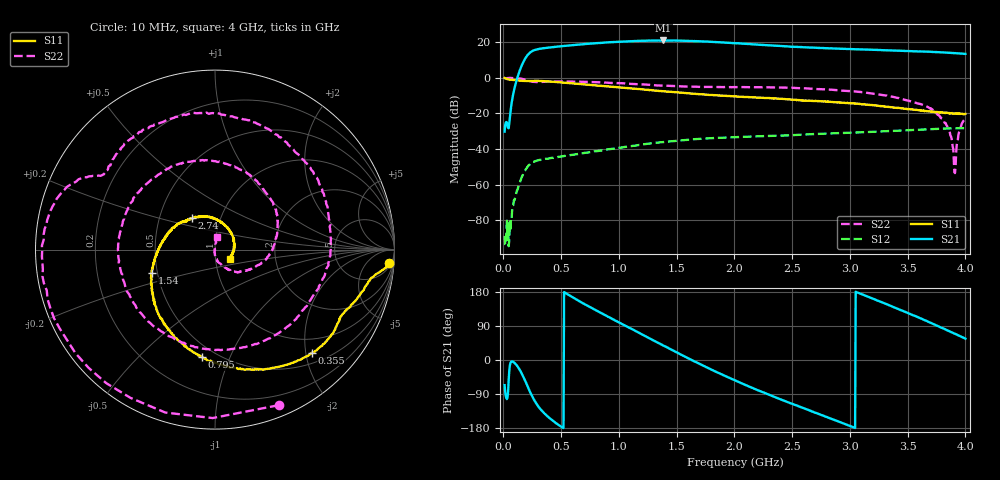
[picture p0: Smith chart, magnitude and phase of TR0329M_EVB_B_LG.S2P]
!Agilent Technologies,E5071C,MY46523237,B.13.01
!Date: Thu Jul 14 13:05:57 2022
!Data & Calibration Information:
!Freq	S11:SOLT2(ON)	S21:SOLT2(ON)	S12:SOLT2(ON)	S22:SOLT2(ON)
!PortZ  Port1:50+j0  Port2:50+j0
!Above PortZ is port z conversion or system Z0 setting when saving the data.
!When reading, reference impedance value at option line is always used.
# Hz S dB R 50
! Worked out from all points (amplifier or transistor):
!   799 points, 10 MHz to 4 GHz, reference 50 ohm
!   highest |S21| = 20.8 dB at 1.385 GHz (marker M1)
!   |S21| within 3 dB of that: 541.7 MHz to 2.374 GHz (1.832 GHz wide, 126 % of centre)
!   unconditionally stable (mu >= 1): start of sweep to end of sweep
!   at 675 MHz: K = 2.45, MAG = 23.8 dB, |S12| = -42.5 dB
!   at 2.005 GHz: K = 1.89, MAG = 20.9 dB, |S12| = -33.4 dB
!   at 4 GHz: K = 2.88, MAG = 13.3 dB, |S12| = -28.3 dB
!   S11 on the Smith chart (normalised r, x): 10 MHz: 9, -23; 355 MHz: 0.70, -2.13; 795 MHz: 0.42, -0.80; 1.54 GHz: 0.47, -0.14; 2.74 GHz: 0.73, +0.27; 4 GHz: 1.17, -0.12
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1e7  -0.25 -4.4  -30.33 -66.4  -88.77 103.1  -0.57 -67.8
1.25e8  -1.59 -20.0  0.84 -18.4  -62.16 -179.2  -0.45 171.6
1.95e8  -1.98 -26.9  11.34 -59.5  -51.30 142.2  -1.36 152.7
2.6e8  -1.90 -33.7  15.18 -102.3  -47.25 103.6  -2.44 146.8
3.55e8  -2.06 -46.6  16.48 -141.1  -45.68 72.9  -2.39 137.9
5.1e8  -2.78 -66.2  17.61 -178.0  -44.06 48.6  -2.22 117.2
6.75e8  -3.73 -84.5  18.60 152.0  -42.49 32.1  -2.42 92.6
7.95e8  -4.38 -96.8  19.20 132.1  -41.37 21.7  -2.61 73.6
1.09e9  -5.96 -124.4  20.31 84.7  -38.57 -4.9  -3.47 21.6
1.34e9  -7.46 -145.3  20.67 45.0  -36.43 -29.7  -4.45 -30.5
1.385e9  -7.70 -148.6  20.78 38.2  -36.19 -34.8  -4.51 -40.4
1.54e9  -8.50 -159.6  20.68 13.4  -35.21 -50.7  -4.94 -75.1
1.745e9  -9.53 -173.2  20.19 -17.0  -34.27 -73.4  -5.27 -120.0
2.005e9  -10.61 171.4  19.25 -53.7  -33.42 -101.0  -5.35 -171.4
2.315e9  -11.60 152.6  18.04 -93.4  -32.69 -132.4  -5.51 137.3
2.67e9  -13.07 131.1  16.77 -135.8  -31.73 -167.1  -6.26 85.6
2.74e9  -13.26 126.6  16.61 -143.5  -31.51 -174.3  -6.53 75.9
3.02e9  -14.42 104.6  15.95 -176.4  -30.90 156.5  -7.68 37.9
3.335e9  -16.47 71.0  15.22 145.1  -30.04 123.0  -10.38 -6.1
3.685e9  -19.03 17.7  14.44 100.0  -28.92 82.7  -16.92 -53.3
3.905e9  -20.17 -17.1  13.68 69.6  -28.48 53.9  -53.07 -81.5
4e9  -20.35 -32.1  13.27 56.4  -28.35 41.1  -22.78 80.7
